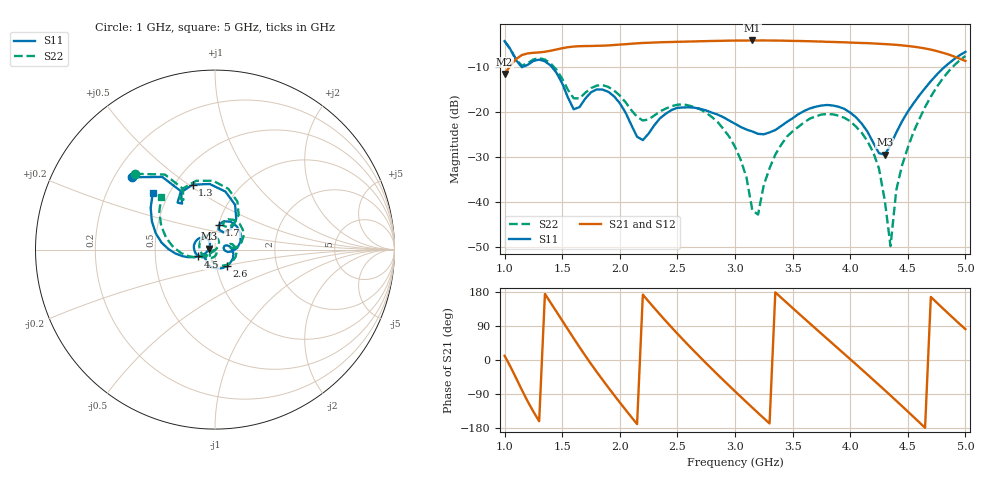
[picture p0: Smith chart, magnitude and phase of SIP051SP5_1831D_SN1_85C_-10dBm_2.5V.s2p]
# GHz  S  dB  R  50
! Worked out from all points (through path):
!   81 points, 1 GHz to 5 GHz, reference 50 ohm
!   highest |S21| = -4.07 dB at 3.15 GHz (marker M1); lowest = -11.5 dB at 1 GHz (marker M2)
!   lowest |S11| = -29.5 dB at 4.3 GHz (marker M3), VSWR 1.07, Z = 46.8 + j0.448 ohm
!   |S11| at or under -10 dB: 1.149155 GHz to 1.1525 GHz (3.345 MHz wide, 0.291 % of centre); 1.411 GHz to 4.819 GHz (3.408 GHz wide, 109 % of centre)
!   |S22| runs from -49.9 to -4.2 dB; largest |S21 - S12| = 0.0022
!   S11 on the Smith chart (normalised r, x): 1 GHz: 0.27, +0.35; 1.3 GHz: 0.61, +0.52; 1.7 GHz: 1.01, +0.28; 2.6 GHz: 1.12, -0.21; 4.5 GHz: 0.83, -0.06; 5 GHz: 0.41, +0.33
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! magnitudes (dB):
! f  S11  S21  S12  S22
! 1 GHz  -4.2  -11.5  -11.5  -4.2
! 1.15 GHz  -10.0  -7.3  -7.3  -9.7
! 1.3 GHz  -8.3  -6.7  -6.7  -8.0
! 1.6 GHz  -19.4  -5.4  -5.4  -17.0
! 1.7 GHz  -17.0  -5.3  -5.3  -15.7
! 1.9 GHz  -15.5  -5.2  -5.2  -14.4
! 2.2 GHz  -26.3  -4.6  -4.6  -21.9
! 2.35 GHz  -21.4  -4.5  -4.5  -19.9
! 2.6 GHz  -18.9  -4.3  -4.3  -18.6
! 3 GHz  -22.6  -4.1  -4.1  -27.8
! 3.15 GHz  -24.3  -4.1  -4.1  -41.9
! 3.2 GHz  -24.9  -4.1  -4.1  -42.8
! 3.4 GHz  -23.1  -4.1  -4.1  -27.3
! 3.7 GHz  -18.8  -4.3  -4.3  -21.0
! 4.1 GHz  -22.6  -4.6  -4.6  -24.6
! 4.25 GHz  -29.2  -4.8  -4.8  -32.6
! 4.3 GHz  -29.5  -4.9  -4.9  -39.6
! 4.35 GHz  -27.4  -5.0  -5.0  -49.9
! 4.4 GHz  -24.6  -5.0  -5.0  -37.4
! 4.5 GHz  -19.9  -5.3  -5.3  -28.0
! 4.75 GHz  -11.7  -6.4  -6.4  -14.5
! 5 GHz  -6.6  -8.6  -8.6  -7.5
